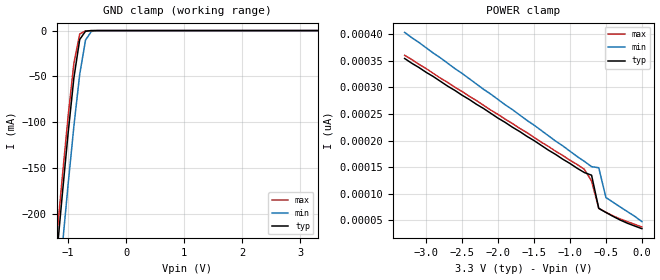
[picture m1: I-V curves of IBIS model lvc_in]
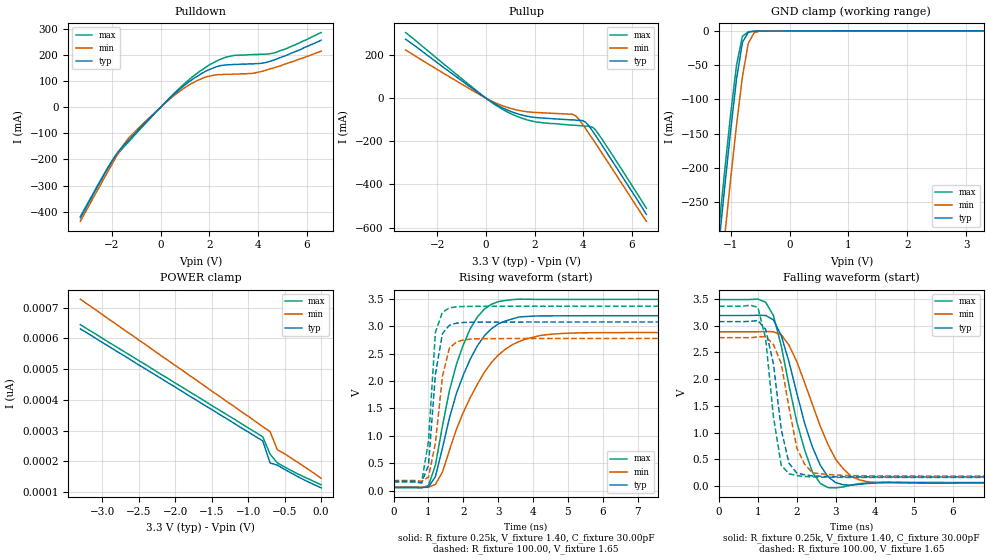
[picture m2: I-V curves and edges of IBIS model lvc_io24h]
| IBIS file 16543xh.ibs created by s2ibis2 version 1.1
| North Carolina State University Electronics Research Laboratory  1995
[IBIS ver]   2.1
[File name]   16543xh.ibs
[File Rev]   1.0
[Date]   03/01/99 rtk rtk
[Source]   Integrated Device Technology, Inc.
[Notes]   1.Temperatures: typ=25C, min=100C, max=0C 2.RRmp rates based
   on 50 ohm load.
[Disclaimer] Integrated Device Technology, Inc. ("IDT") hereby grants the
   user of this IBIS model a non-exclusive, nontransferable
   license to use this IBIS model under the following terms. The
   user is granted this license only to use the IBIS model and is
   not granted rights to sell, copy (except as needed to run the
   IBIS model), rent, lease or sub-license the IBIS model in
   whole or in part, or in modified form to anyone. The User may
   modify the IBIS model to suit its specific applications, but
   rights to derivative works and such modifications shall belong
   to IDT. This IBIS model is provided on an AS IS" basis and IDT
   makes absolutely no warranty with respect to the information
   contained herein. IDT DISCLAIMS AND CUSTOMER WAIVES ALL
   WARRANTIES, EXPRESS AND IMPLIED, INCLUDING WARRANTIES OF
   MERCHANTABILITY AND FITNESS FOR A PARTICULAR PURPOSE. THE
   ENTIRE RISK AS TO QUALITY AND PERFORMANCE IS WITH THE USER
   ACCORDINGLY, IN NO EVENT SHALL IDT BE LIABLE FOR ANY DIRECT OR
   INDIRECT DAMAGES, WHETHER IN CONTRACT OR TORT, INCLUDING ANY
   LOST PROFITS OR OTHER INCIDENTAL, CONSEQUENTIAL, EXEMPLARY, OR
   PUNITIVE DAMAGES ARISING OUT OF THE USE OR APPLICATION OF THE
   IBIS model. Further, IDT reserves the right to make changes
   without notice to any product herein to improve reliability,
   function, or design. IDT does not convey any license under
   patent rights or any other intellectual property rights,
   including those of third parties. IDT is not obligated to
   provide maintenance or support for the licensed IBIS model.
[Copyright]   Copyright 1997, Integrated Device Technology, Inc. all rights
   reserved
|   Component LVCH16543
[Component]   LVCH16543
[Manufacturer]   Integrated Device Technology
[Package]
| PA56
| variable   typ   min   max
R_pkg   6.50m   5.00m   10.00m
L_pkg   3.30nH   2.50nH   4.90nH
C_pkg   0.29pF   0.010pF   1.16pF
[Pin]  signal_name   model_name   R_pin   L_pin   C_pin
1   1OEAB_   lvc_in
2   1LEAB_   lvc_in
3   1CEAB_   lvc_in
4   GND   GND
5   1A1   lvc_io24h
6   1A2   lvc_io24h
7   VCC   POWER
8   1A3   lvc_io24h
9   1A4   lvc_io24h
10   1A5   lvc_io24h
11   GND   GND
12   1A6   lvc_io24h
13   1A7   lvc_io24h
14   1A8   lvc_io24h
15   2A1   lvc_io24h
16   2A2   lvc_io24h
17   2A3   lvc_io24h
18   GND   GND
19   2A4   lvc_io24h
20   2A5   lvc_io24h
21   2A6   lvc_io24h
22   VCC   POWER
23   2A7   lvc_io24h
24   2A8   lvc_io24h
25   GND   GND
26   2CEAB_   lvc_in
27   2LEAB_   lvc_in
28   2OEAB_   lvc_in
29   2OEBA_   lvc_in
30   2LEBA_   lvc_in
31   2CEBA_   lvc_in
32   GND   GND
33   2B8   lvc_io24h
34   2B7   lvc_io24h
35   VCC   POWER
36   2B6   lvc_io24h
37   2B5   lvc_io24h
38   2B4   lvc_io24h
39   GND   GND
40   2B3   lvc_io24h
41   2B2   lvc_io24h
42   2B1   lvc_io24h
43   1B8   lvc_io24h
44   1B7   lvc_io24h
45   1B6   lvc_io24h
46   GND   GND
47   1B5   lvc_io24h
48   1B4   lvc_io24h
49   1B3   lvc_io24h
50   VCC   POWER
51   1B2   lvc_io24h
52   1B1   lvc_io24h
53   GND   GND
54   1CEBA_   lvc_in
55   1LEBA_   lvc_in
56   1OEBA_   lvc_in
| Models and submodels in the file (2): lvc_in (Input), lvc_io24h (I/O)
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| in   in   dummy_model
| oe   oe
|   Model lvc_in
[Model]   lvc_in
Model_type   Input
Vinl =  0.800V
Vinh =  2.000V
C_comp   3.00pF   NA   NA
[Temperature Range]   25.00   100.00   0.000
[Voltage Range]   3.30V   3.00V   3.60V
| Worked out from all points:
|   GND clamp passes 1 mA (typ) near -0.70 V on its own axis
[GND_clamp]
| voltage   I(typ)   I(min)   I(max)
-3.3V     -1.806A    -1.858A    -1.789A
-1.2V     -248mA     -306mA     -229mA
-1.1V     -179mA     -236mA     -160mA
-1V       -112mA     -168mA     -93.56mA
-900mV    -51.39mA   -104mA     -35.36mA
-800mV    -9.697mA   -47.7mA    -3.786mA
-700mV    -714uA     -10.4mA    -348uA
-600mV    -52.42uA   -951uA     -8.225uA
-500mV    -126nA     -30.48uA   -10.89nA
3.3V      34.69pA    75.27pA    23pA
[POWER_clamp]
| voltage   I(typ)   I(min)   I(max)
-3.3V     354pA      403pA      360pA
-800mV    140pA      161pA      146pA
-700mV    135pA      151pA      124pA
-600mV    72.75pA    149pA      72.79pA
-500mV    65.09pA    93.05pA    65.39pA
-300mV    50.77pA    75.27pA    52.78pA
0V        34.68pA    47.91pA    37.83pA
|   Model lvc_io24h
[Model]   lvc_io24h
Model_type   I/O
Polarity   Non-Inverting
Enable   Active-High
Vinl =  0.000V
Vinh =  2.000V
Vmeas =  1.500V
C_comp   3.00pF   NA   NA
[Temperature Range]   25.00   100.00   0.000
[Voltage Range]   3.30V   3.00V   3.60V
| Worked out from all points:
|   slope of the pulldown table from 0 to 0.495 V, typ, clamps not added: 11.1 ohm
|   slope of the pullup table from 0 to 0.495 V, typ, clamps not added: 14.5 ohm
|   GND clamp passes 1 mA (typ) near -0.64 V on its own axis
|   rising waveform, R_fixture 0.25k, V_fixture 1.40, C_fixture 30.00pF: 20-80 % time 974ps typ, 1.24ns min, 819ps max; typ from 0.061 V to 3.19 V
|   rising waveform, R_fixture 100.00, V_fixture 1.65: 20-80 % time 266ps typ, 323ps min, 208ps max; typ from 0.171 V to 3.08 V
|   falling waveform, R_fixture 0.25k, V_fixture 1.40, C_fixture 30.00pF: 20-80 % time 725ps typ, 902ps min, 639ps max; typ from 3.19 V to 0.061 V
|   falling waveform, R_fixture 100.00, V_fixture 1.65: 20-80 % time 362ps typ, 397ps min, 304ps max; typ from 3.08 V to 0.171 V
[Pulldown]
| voltage   I(typ)   I(min)   I(max)
-3.3V     -424mA     -437mA     -419mA
-2.1V     -223mA     -235mA     -220mA
-1.8V     -177mA     -186mA     -182mA
-1.4V     -135mA     -128mA     -141mA
47.68nV   4.51nA     4.11nA     4.76nA
900mV     77.7mA     68.8mA     83.4mA
1.8V      135mA      114mA      150mA
2.6V      161mA      126mA      189mA
3.7V      166mA      129mA      201mA
4.4V      173mA      144mA      204mA
5.1V      196mA      165mA      222mA
6.6V      257mA      215mA      286mA
[Pullup]
| voltage   I(typ)   I(min)   I(max)
-3.3V     273mA      223mA      304mA
-200mV    15.7mA     12.6mA     17.8mA
800mV     -51.2mA    -39.9mA    -59.2mA
1.4V      -75.9mA    -58mA      -89.7mA
2V        -89.2mA    -66.1mA    -109mA
3.5V      -101mA     -74.3mA    -125mA
3.7V      -102mA     -83mA      -126mA
4.1V      -112mA     -141mA     -130mA
4.4V      -155mA     -191mA     -136mA
4.5V      -172mA     -208mA     -147mA
5.2V      -292mA     -329mA     -263mA
6.6V      -539mA     -571mA     -511mA
[GND_clamp]
| voltage   I(typ)   I(min)   I(max)
-3.3V     -2.217A    -2.283A    -2.195A
-1.2V     -312mA     -384mA     -288mA
-1.1V     -227mA     -299mA     -203mA
-1V       -145mA     -216mA     -121mA
-900mV    -69.9mA    -137mA     -49.49mA
-800mV    -16.48mA   -66.49mA   -7.75mA
-700mV    -2.021mA   -17.86mA   -1.171mA
-600mV    -313uA     -2.437mA   -215uA
-500mV    -136uA     -188uA     -155uA
3.3V      163uA      116uA      211uA
[POWER_clamp]
| voltage   I(typ)   I(min)   I(max)
-3.3V     631pA      728pA      645pA
-800mV    267pA      313pA      280pA
-700mV    195pA      297pA      224pA
-600mV    188pA      238pA      195pA
-300mV    148pA      194pA      157pA
0V        114pA      145pA      124pA
[Ramp]
| variable   typ   min   max
dV/dt_r   1.45/0.32n   1.21/0.34n   1.64/0.23n
dV/dt_f   1.59/0.39n   1.41/0.50n   1.76/0.35n
R_load = 50.00
[Rising Waveform]
R_fixture = 0.25k
V_fixture = 1.40
C_fixture = 30.00pF
R_dut = 7.00m
L_dut = 3.30nH
C_dut = 0.29pF
| time   V(typ)   V(min)   V(max)
0s        61.18mV    67.45mV    57.75mV
1ns       68.22mV    64.57mV    94.91mV
1.2ns     260mV      117mV      469mV
1.4ns     775mV      340mV      1.176V
1.6ns     1.324V     733mV      1.82V
2ns       2.108V     1.429V     2.659V
2.4ns     2.635V     1.936V     3.163V
3ns       3.038V     2.47V      3.444V
5ns       3.187V     2.869V     3.484V
19.8ns    3.189V     2.884V     3.487V
[Rising Waveform]
R_fixture = 100.00
V_fixture = 1.65
R_dut = 7.00m
L_dut = 3.30nH
C_dut = 0.29pF
| time   V(typ)   V(min)   V(max)
0s        171mV      188mV      161mV
800ps     147mV      174mV      143mV
1ns       463mV      248mV      895mV
1.2ns     2.124V     874mV      2.888V
1.4ns     2.86V      2.079V     3.252V
1.6ns     3.014V     2.598V     3.329V
1.8ns     3.052V     2.708V     3.35V
2ns       3.065V     2.747V     3.356V
2.6ns     3.071V     2.77V      3.359V
19.8ns    3.075V     2.775V     3.362V
[Falling Waveform]
R_fixture = 0.25k
V_fixture = 1.40
C_fixture = 30.00pF
R_dut = 7.00m
L_dut = 3.30nH
C_dut = 0.29pF
| time   V(typ)   V(min)   V(max)
0s        3.189V     2.884V     3.487V
1ns       3.194V     2.885V     3.495V
1.4ns     3.106V     2.884V     3.187V
1.8ns     2.32V      2.633V     1.883V
2.2ns     1.176V     1.933V     680mV
2.4ns     732mV      1.53V      262mV
2.8ns     175mV      780mV      -28.91mV
3.4ns     17.82mV    181mV      19.19mV
4ns       57.02mV    65.71mV    68.19mV
19.8ns    61.19mV    67.46mV    57.75mV
[Falling Waveform]
R_fixture = 100.00
V_fixture = 1.65
R_dut = 7.00m
L_dut = 3.30nH
C_dut = 0.29pF
| time   V(typ)   V(min)   V(max)
0s        3.075V     2.775V     3.362V
1ns       3.095V     2.788V     3.342V
1.2ns     2.931V     2.794V     2.759V
1.4ns     2.285V     2.647V     1.295V
1.6ns     1.061V     2.291V     390mV
1.8ns     428mV      1.467V     231mV
2ns       243mV      713mV      198mV
2.4ns     193mV      248mV      172mV
3.2ns     174mV      201mV      163mV
19.8ns    171mV      188mV      161mV
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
